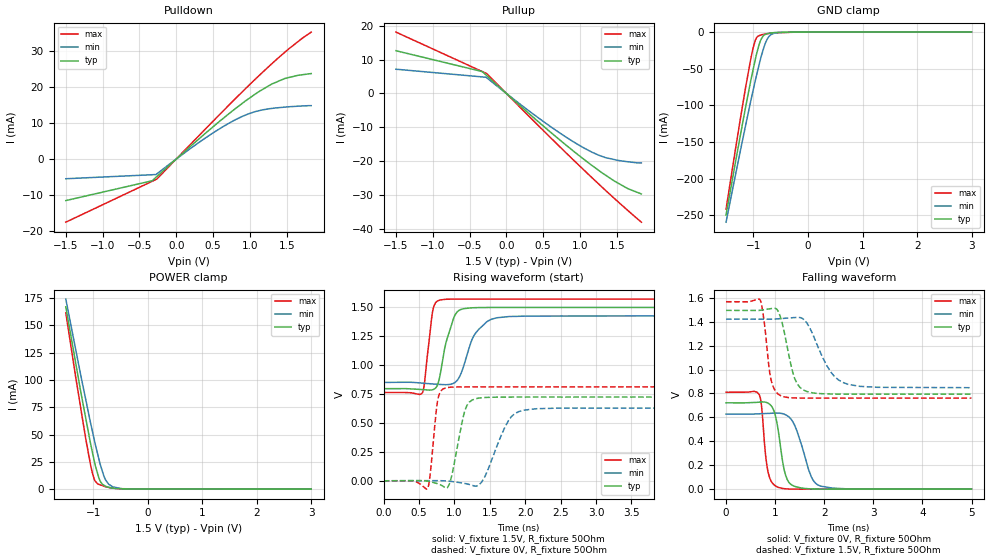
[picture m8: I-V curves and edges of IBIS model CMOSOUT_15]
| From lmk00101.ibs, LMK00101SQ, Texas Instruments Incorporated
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|   Model CMOSOUT_15
[Model]   CMOSOUT_15
Model_type   3-state
Polarity   Non-Inverting
Vmeas = .75
Vref = .75
Cref = 15pF
Rref = 50
|   typ   min   max
|   Nom   Strong   Weak
C_comp   0.4977p   0.4681p   0.5375p
|Output in High
|C_Comp high   0.4977p   0.4681p   0.5375p
|Output in low
|C_Comp low   0.9197p   0.9197p   0.9197p
|Output disabled
|C_Comp disabled   0.8920p   0.8648p   0.9197p
[Voltage Range]   1.5   1.425   1.575
[Temperature Range]   45   125   -40
[Pullup Reference]   1.5   1.425   1.575
[Pulldown Reference]   0   0   0
[Power Clamp Reference]   1.5   1.425   1.575
[GND Clamp Reference]   0   0   0
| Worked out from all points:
|   slope of the pulldown table from 0 to 0.225 V, typ, clamps not added: 54.6 ohm
|   slope of the pullup table from 0 to 0.225 V, typ, clamps not added: 51.6 ohm
|   GND clamp passes 1 mA (typ) near -0.66 V on its own axis
|   POWER clamp passes 1 mA (typ) near -0.65 V on its own axis
|   falling waveform, V_fixture 0V, R_fixture 50Ohm: 20-80 % time 170ps typ, 287ps min, 114ps max; typ from 0.722 V to 0 V
|   rising waveform, V_fixture 1.5V, R_fixture 50Ohm: 20-80 % time 160ps typ, 229ps min, 87.8ps max; typ from 0.794 V to 1.5 V
|   rising waveform, V_fixture 0V, R_fixture 50Ohm: 20-80 % time 140ps typ, 256ps min, 76.2ps max; typ from 0 V to 0.722 V
|   falling waveform, V_fixture 1.5V, R_fixture 50Ohm: 20-80 % time 228ps typ, 412ps min, 138ps max; typ from 1.5 V to 0.794 V
[Pulldown]
|   Voltage   I(typ)   I(min)   I(max)
-1.5V     -11.58mA   -5.497mA   -17.61mA
-326.7mV  -6.062mA   -4.38mA    -6.206mA
-263.7mV  -4.891mA   -4.145mA   -5.594mA
174.6mV   3.192mA    2.659mA    3.696mA
444.6mV   8.013mA    6.531mA    9.377mA
714.6mV   12.61mA    9.967mA    15mA
894.6mV   15.48mA    11.86mA    18.68mA
1.075V    18.11mA    13.23mA    22.27mA
1.293V    20.86mA    14.09mA    26.47mA
1.473V    22.44mA    14.46mA    29.74mA
1.653V    23.33mA    14.72mA    32.72mA
1.833V    23.82mA    14.87mA    35.38mA
[GND Clamp]
|   Voltage   I(typ)   I(min)   I(max)
-1.5V     -249.5mA   -259.4mA   -241.8mA
-1.317V   -173.1mA   -191mA     -154.8mA
-1.137V   -100.4mA   -125.5mA   -73.32mA
-1.047V   -66.05mA   -93.86mA   -36.5mA
-990.4mV  -46.41mA   -74.93mA   -17.69mA
-939.7mV  -29.47mA   -58.49mA   -7.615mA
-857.2mV  -9.66mA    -33.52mA   -3.826mA
-769.1mV  -2.772mA   -13.16mA   -2.419mA
-679.1mV  -1.156mA   -3.604mA   -1.494mA
-545.4mV  -486.8uA   -562.5uA   -773uA
-275.4mV  -144.9uA   -99.29uA   -225.8uA
2.995V    0A         0A         0A
[Pullup]
|   Voltage   I(typ)   I(min)   I(max)
-1.5V     12.59mA    7.143mA    18.07mA
-326.7mV  6.441mA    4.872mA    6.437mA
-263.7mV  5.194mA    4.567mA    5.812mA
174.6mV   -3.38mA    -2.945mA   -3.822mA
534.6mV   -10.19mA   -8.751mA   -11.61mA
804.6mV   -15.09mA   -12.77mA   -17.35mA
1.075V    -19.75mA   -16.3mA    -22.99mA
1.345V    -24.01mA   -18.88mA   -28.48mA
1.473V    -25.87mA   -19.49mA   -31.04mA
1.653V    -28.06mA   -20.11mA   -34.52mA
1.833V    -29.58mA   -20.47mA   -37.9mA
[POWER Clamp]
|   Voltage   I(typ)   I(min)   I(max)
-1.5V     167mA      174.1mA    161.5mA
-1.317V   115mA      127.4mA    102mA
-1.137V   65.55mA    82.58mA    46.7mA
-1.047V   41.7mA     60.71mA    22.29mA
-1.013V   33.91mA    53.03mA    14.8mA
-962.2mV  22.22mA    41.5mA     7.354mA
-868.5mV  7.24mA     22.49mA    3.91mA
-780.3mV  2.996mA    9.405mA    2.409mA
-712.8mV  1.717mA    4.451mA    1.561mA
-634.1mV  905.9uA    2.013mA    1.007mA
-455.4mV  379.5uA    226.4uA    393.9uA
2.995V    0A         0A         0A
[Ramp]
R_load = 50
|   typ   min   max
dV/dt_r   0.420369/1.59621e-10   0.343949/2.2898e-10   0.483596/8.76463e-11
dV/dt_f   0.433239/1.6919e-10   0.376567/2.834e-10   0.486016/1.1287e-10
[Falling Waveform]
V_fixture = 0V
V_fixture_min = 0V
V_fixture_max = 0V
R_fixture = 50Ohm
C_fixture = 0F
|   Time   V(typ)   V(min)   V(max)
0s        722.1mV    627.6mV    810mV
674ps     727.3mV    630.3mV    792.5mV
722ps     729.2mV    631.1mV    698.9mV
855ps     719.3mV    633.3mV    145.5mV
1.063ns   490.3mV    636.4mV    15.67mV
1.18ns    170mV      627.6mV    4.418mV
1.285ns   54.47mV    602.1mV    1.336mV
1.737ns   2.203mV    102.6mV    10.17uV
1.93ns    505.5uV    24.91mV    1.721uV
4.999ns   5.669nV    116.8nV    5.72nV
[Rising Waveform]
V_fixture = 1.5V
V_fixture_min = 1.425V
V_fixture_max = 1.575V
R_fixture = 50Ohm
C_fixture = 0F
|   Time   V(typ)   V(min)   V(max)
0s        794.2mV    848.4mV    761.2mV
547ps     786.6mV    842.1mV    758.8mV
693ps     785.3mV    835mV      1.464V
794ps     902.2mV    831mV      1.558V
876ps     1.18V      828.7mV    1.565V
984ps     1.394V     839.4mV    1.567V
1.121ns   1.483V     971.7mV    1.567V
1.289ns   1.493V     1.266V     1.567V
1.598ns   1.495V     1.406V     1.567V
4.999ns   1.495V     1.422V     1.567V
[Rising Waveform]
V_fixture = 0V
V_fixture_min = 0V
V_fixture_max = 0V
R_fixture = 50Ohm
C_fixture = 0F
|   Time   V(typ)   V(min)   V(max)
0s        5.634nV    29.97nV    5.72nV
619ps     -2.945mV   1.024mV    -69.84mV
654ps     -7.203mV   1.024mV    38.53mV
763ps     -25.85mV   984.2uV    694.1mV
878ps     -62.56mV   -1.398mV   800.9mV
955ps     27.22mV    -5.967mV   807.5mV
1.151ns   611.1mV    -23.49mV   809.9mV
1.287ns   705.1mV    -45.66mV   810mV
1.907ns   721.9mV    596.2mV    810mV
4.999ns   722mV      627.6mV    810mV
[Falling Waveform]
|Gnd
V_fixture = 1.5V
V_fixture_min = 1.425V
V_fixture_max = 1.575V
R_fixture = 50Ohm
C_fixture = 0F
|   Time   V(typ)   V(min)   V(max)
0s        1.495V     1.422V     1.567V
694ps     1.496V     1.421V     1.583V
762ps     1.5V       1.421V     1.444V
914ps     1.509V     1.421V     919.4mV
1.134ns   1.402V     1.427V     777.9mV
1.395ns   929mV      1.435V     762.7mV
1.614ns   821.8mV    1.407V     761.4mV
2.048ns   796.6mV    1.036V     761.2mV
2.375ns   794.6mV    893mV      761.2mV
4.999ns   794.2mV    848.4mV    761.2mV
